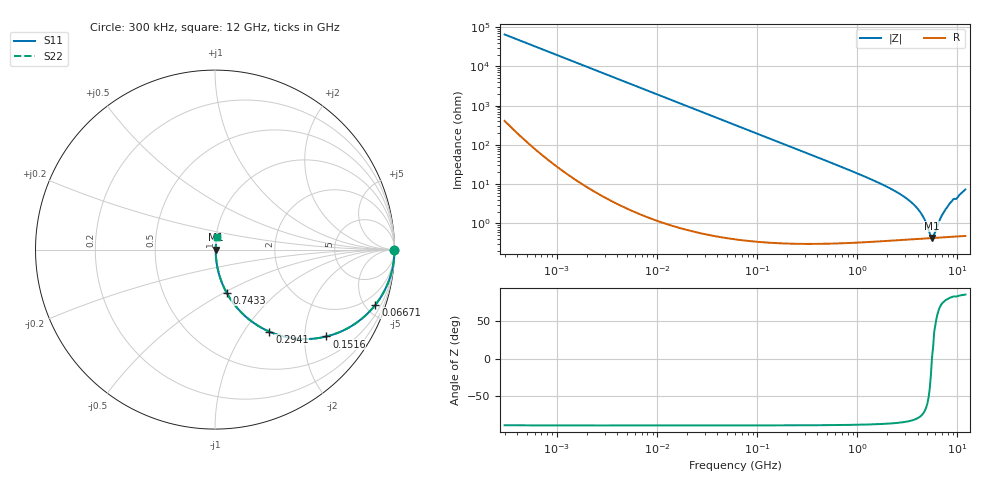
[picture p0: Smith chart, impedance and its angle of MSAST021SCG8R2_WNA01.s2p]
! MSAST021SCG8R2_WNA01  S-PARAMETER MODEL  ( General Type )
! Model Generated by TAIYO YUDEN Corporation (http://www.ty-top.com)
! Version 2.0
! TAIYO YUDEN Control No. 181101
! Copyright(c) 2015 TAIYO YUDEN CO.,LTD. All Rights Reserved.
! Product Description (link to TY-COMPAS)
! https://ds.yuden.co.jp/TYCOMPAS/or/detail?pn=MSAST021SCG8R2CWNA01&u=M
! Products Name : Multilayer Ceramic Capacitors
! Characteristics :
!  Capacitance : 8.2 pF , Rated Voltage : 25V , TCC : CG / C0G
!  Case Size : 0.25 x 0.125 / 0.0098 x 0.0049 [mm/inch] , Thickness : 0.125 / 0.0049 [mm/inch]
!  (Conditions: Temperature = 25 degC , DC Bias Current/Voltage = 0A / 0V)
! External Node Assignments :
!  1  o---| |---o  2
! GND o---------o GND
! Frequency Range : 0.3MHz  -  12000MHz  [ 401 STEP ]
# MHz S RI R 50
! Freq[MHz].  S11 Real  S11 Imag  S21 Real  S21 Imag  S12 Real  S12 Imag  S22 Real  S22 Imag
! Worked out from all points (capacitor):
!   401 points, 300 kHz to 12 GHz, reference 50 ohm
!   read as one part in series: C = 8.2 pF near 316.3 kHz
!   lowest |Z| = 428 mohm at 5.566 GHz (marker M1)
!   series resonance near 5.561 GHz, so ESL is about 100 pH
!   S11 on the Smith chart (normalised r, x): 300 kHz: open; 66.71 MHz: 1.01, -5.82; 151.6 MHz: 1.01, -2.56; 294.1 MHz: 1.01, -1.32; 743.3 MHz: 1.01, -0.51; 12 GHz: 1.01, +0.15
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0.3  1 -0.00155  1.21e-05 0.00155  1.21e-05 0.00155  1 -0.00155
1.769972  0.9999 -0.00912  9.16e-05 0.00912  9.16e-05 0.00912  0.9999 -0.00912
10.44266  0.9971 -0.0536  0.00292 0.0536  0.00292 0.0536  0.9971 -0.0536
27.10171  0.9808 -0.1369  0.0192 0.1369  0.0192 0.1369  0.9808 -0.1369
60  0.9125 -0.282  0.0875 0.282  0.0875 0.282  0.9125 -0.282
66.70707  0.894 -0.3072  0.106 0.3072  0.106 0.3072  0.894 -0.3072
99.25425  0.7922 -0.4049  0.2078 0.4049  0.2078 0.4049  0.7922 -0.4049
151.6462  0.6203 -0.4841  0.3797 0.4841  0.3797 0.4841  0.6203 -0.4841
294.0765  0.3031 -0.4573  0.6969 0.4573  0.6969 0.4573  0.3031 -0.4573
353.9943  0.231 -0.4187  0.769 0.4187  0.769 0.4187  0.231 -0.4187
743.2595  0.0643 -0.2392  0.9357 0.2392  0.9357 0.2392  0.0643 -0.2392
2088.533  0.00988 -0.0788  0.9901 0.0788  0.9901 0.0788  0.00988 -0.0788
3026.31  0.00586 -0.0447  0.9941 0.0447  0.9941 0.0447  0.00586 -0.0447
3841.137  0.0047 -0.0262  0.9953 0.0262  0.9953 0.0262  0.0047 -0.0262
4502.883  0.00434 -0.0148  0.9957 0.0148  0.9957 0.0148  0.00434 -0.0148
5278.635  0.00424 -0.00367  0.9958 0.00367  0.9958 0.00367  0.00424 -0.00367
5565.855  0.00426 6.58e-05  0.9957 -6.58e-05  0.9957 -6.58e-05  0.00426 6.58e-05
5868.704  0.00431 0.0032  0.9957 -0.0032  0.9957 -0.0032  0.00431 0.0032
6879.757  0.00461 0.0141  0.9954 -0.0141  0.9954 -0.0141  0.00461 0.0141
8064.993  0.00528 0.0275  0.9947 -0.0275  0.9947 -0.0275  0.00528 0.0275
8732.115  0.00584 0.0354  0.9942 -0.0354  0.9942 -0.0354  0.00584 0.0354
12000  0.0101 0.0722  0.9899 -0.0722  0.9899 -0.0722  0.0101 0.0722
